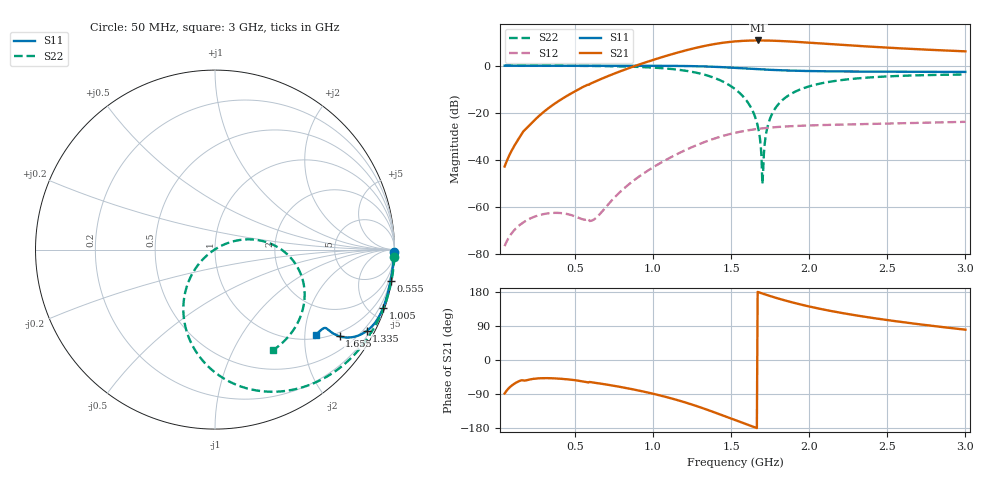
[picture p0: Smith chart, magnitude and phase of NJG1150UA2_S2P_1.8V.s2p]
!	Created	Tue	Apr	17	16:25:33	2012
#	hz	S	ma	R	50
!	2	Port	Network	Data	from	SP1.SP	block
!	freq	magS11	angS11	magS21	angS21	magS12	angS12	magS22	angS22
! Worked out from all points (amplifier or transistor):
!   591 points, 50 MHz to 3 GHz, reference 50 ohm
!   highest |S21| = 10.7 dB at 1.675 GHz (marker M1)
!   |S21| within 3 dB of that: 1.284 GHz to 2.488 GHz (1.205 GHz wide, 63.9 % of centre)
!   unconditionally stable (mu >= 1): 544.1 MHz to end of sweep
!   at 540 MHz: K = 0.95, MSG = 27.8 dB, |S12| = -65.0 dB
!   at 1.525 GHz: K = 1.03, MAG = 18.3 dB, |S12| = -28.5 dB
!   at 3 GHz: K = 1.31, MAG = 11.6 dB, |S12| = -23.8 dB
!   lowest NFmin = 0.22 dB at 525 MHz
!   S11 on the Smith chart (normalised r, x): 50 MHz: open; 555 MHz: 0, -11; 1.005 GHz: 0.16, -5.89; 1.335 GHz: 0.35, -3.94; 1.655 GHz: 0.87, -2.95; 3 GHz: 1.11, -2.28
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5e7  0.9964 -0.9  0.007251 -88.5  0.0001484 88.4  0.9999 -2.3
1.3e8  0.9961 -2.3  0.02493 -58.3  0.0003733 87.4  0.9994 -6.1
2.55e8  0.9953 -4.6  0.07696 -48.8  0.0006488 86.9  0.9977 -12.0
5.45e8  0.9935 -9.9  0.3434 -55.9  0.0005575 117.0  0.9869 -26.9
5.55e8  0.9935 -10.1  0.3569 -56.5  0.0005459 121.7  0.9862 -27.4
6.3e8  0.993 -11.5  0.4598 -60.1  0.00057 164.5  0.9814 -31.7
1.005e9  0.9913 -19.3  1.334 -89.5  0.007116 -154.4  0.9056 -58.3
1.035e9  0.9906 -20.0  1.434 -92.5  0.008155 -155.9  0.8928 -61.0
1.185e9  0.9826 -23.9  2.001 -109.3  0.01492 -166.8  0.7988 -76.3
1.335e9  0.9589 -28.3  2.633 -129.5  0.0243 177.9  0.6349 -95.1
1.43e9  0.9318 -30.9  2.994 -143.8  0.03104 166.4  0.4889 -108.5
1.525e9  0.8967 -33.1  3.259 -158.6  0.03754 154.2  0.3187 -122.6
1.655e9  0.8457 -34.9  3.412 -178.2  0.04478 137.9  0.07962 -141.9
1.675e9  0.8385 -35.0  3.415 178.9  0.04568 135.6  0.04491 -145.3
1.695e9  0.8316 -35.1  3.413 176.1  0.04651 133.3  0.01117 -152.7
1.705e9  0.8282 -35.2  3.41 174.7  0.04691 132.2  0.005549 45.1
1.73e9  0.8202 -35.3  3.4 171.4  0.04783 129.4  0.04553 30.7
1.78e9  0.8059 -35.4  3.362 164.9  0.04944 124.2  0.1203 23.6
2.02e9  0.7648 -35.2  3.033 139.4  0.05411 104.1  0.3796 -1.0
2.23e9  0.751 -35.5  2.725 122.6  0.0564 91.7  0.5044 -17.1
2.51e9  0.743 -36.7  2.395 104.8  0.05908 79.5  0.5921 -34.3
3e9  0.7346 -40.1  2.006 80.0  0.06427 63.4  0.6474 -60.2
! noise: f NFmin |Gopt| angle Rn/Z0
5e+07  0.4621  0.9577  2.387  3.522
3.75e+08  0.2384  0.9023  6.352  0.8308
7.05e+08  0.2376  0.8663  10.52  0.5644
1.03e+09  0.2888  0.8376  14.67  0.5027
1.36e+09  0.357  0.8088  18.95  0.4742
1.685e+09  0.432  0.7804  23.17  0.4556
2.015e+09  0.5124  0.7516  27.43  0.44
2.34e+09  0.5952  0.7235  31.6  0.4261
2.67e+09  0.6823  0.6957  35.78  0.4132
3e+09  0.7737  0.669  39.87  0.4021
